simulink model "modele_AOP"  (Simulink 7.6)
settings: Solver=ode45  StartTime=0.0  StopTime=10.0  RelTol=1e-3
InitFcn:
  | Ad=10^5;
  | Vsat=15;
libraries: fl_lib x18

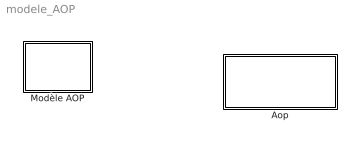
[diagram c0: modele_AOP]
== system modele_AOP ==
  Aop : Subsystem
  Modèle AOP : Subsystem

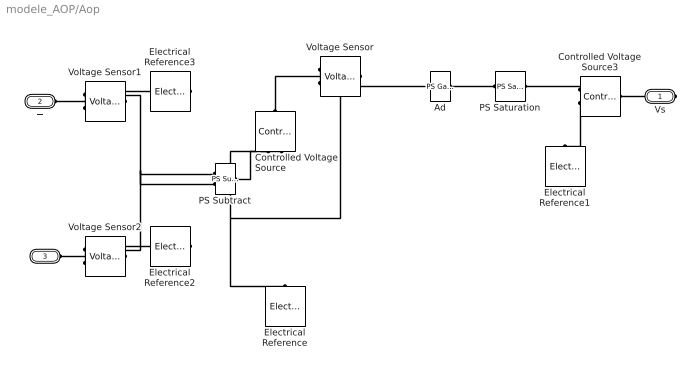
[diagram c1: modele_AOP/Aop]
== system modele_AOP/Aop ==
  Ad : fl_lib/Physical Signals/Functions/PS Gain  DialogController=NetworkEngine.DynNeDlgSource  SystemSampleTime=-1  gain=Ad  LocalVarLogging=[]
  Controlled Voltage Source : fl_lib/Electrical/Electrical Sources/Controlled Voltage Source  DialogController=NetworkEngine.DynNeDlgSource  SystemSampleTime=-1  i_Log=off  v_Log=off  LocalVarNames=|i|v  LocalVarDescs=|i|v  LocalVarLogging=[0 0]
  Controlled Voltage Source3 : fl_lib/Electrical/Electrical Sources/Controlled Voltage Source  DialogController=NetworkEngine.DynNeDlgSource  SystemSampleTime=-1  i_Log=off  v_Log=off  LocalVarNames=|i|v  LocalVarDescs=|i|v  LocalVarLogging=[0 0]
  Electrical Reference{,1..3} (4 alike) : fl_lib/Electrical/Electrical Elements/Electrical Reference  DialogController=NetworkEngine.DynNeDlgSource  SystemSampleTime=-1  i_Log=off  LocalVarNames=|i  LocalVarDescs=|i  LocalVarLogging=0
  PS Saturation : fl_lib/Physical Signals/Nonlinear Operators/PS Saturation  DialogController=NetworkEngine.DynNeDlgSource  SystemSampleTime=-1  upper_limit=Vsat  lower_limit=-Vsat  LocalVarLogging=[]
  PS Subtract : fl_lib/Physical Signals/Functions/PS Subtract  DialogController=NetworkEngine.DynNeDlgSource  SystemSampleTime=-1  LocalVarLogging=[]
  Voltage Sensor : fl_lib/Electrical/Electrical Sensors/Voltage Sensor  DialogController=NetworkEngine.DynNeDlgSource  SystemSampleTime=-1  i1_Log=off  v1_Log=off  LocalVarNames=|i1|v1  LocalVarDescs=|i1|v1  LocalVarLogging=[0 0]
  Voltage Sensor1 : fl_lib/Electrical/Electrical Sensors/Voltage Sensor  DialogController=NetworkEngine.DynNeDlgSource  SystemSampleTime=-1  i1_Log=off  v1_Log=off  LocalVarNames=|i1|v1  LocalVarDescs=|i1|v1  LocalVarLogging=[0 0]
  Voltage Sensor2 : fl_lib/Electrical/Electrical Sensors/Voltage Sensor  DialogController=NetworkEngine.DynNeDlgSource  SystemSampleTime=-1  i1_Log=off  v1_Log=off  LocalVarNames=|i1|v1  LocalVarDescs=|i1|v1  LocalVarLogging=[0 0]
  Vs : PMIOPort  Port=1  Side=Right
  + : PMIOPort  Port=2  Side=Left
  - : PMIOPort  Port=3  Side=Left
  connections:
  Voltage Sensor/RConn1 -- Ad/LConn1
  PS Saturation/LConn1 -- Ad/RConn1
  Controlled Voltage Source/LConn1 -- Voltage Sensor/LConn1
  PS Subtract/RConn1 -- Controlled Voltage Source/RConn1
  Voltage Sensor/RConn2 -- Electrical Reference/LConn1 -- Controlled Voltage Source/RConn2
  Controlled Voltage Source3/RConn1 -- PS Saturation/RConn1
  Controlled Voltage Source3/RConn2 -- Electrical Reference1/LConn1
  Vs/RConn1 -- Controlled Voltage Source3/LConn1
  +/RConn1 -- Voltage Sensor1/LConn1
  -/RConn1 -- Voltage Sensor2/LConn1
  Voltage Sensor2/RConn1 -- PS Subtract/LConn2
  Voltage Sensor1/RConn1 -- PS Subtract/LConn1
  Voltage Sensor1/RConn2 -- Electrical Reference3/LConn1
  Voltage Sensor2/RConn2 -- Electrical Reference2/LConn1

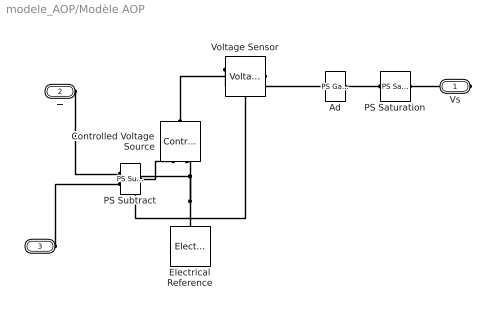
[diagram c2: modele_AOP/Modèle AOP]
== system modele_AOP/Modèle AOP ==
  Ad : fl_lib/Physical Signals/Functions/PS Gain  DialogController=NetworkEngine.DynNeDlgSource  SystemSampleTime=-1  gain=Ad  LocalVarLogging=[]
  Controlled Voltage Source : fl_lib/Electrical/Electrical Sources/Controlled Voltage Source  DialogController=NetworkEngine.DynNeDlgSource  SystemSampleTime=-1  i_Log=off  v_Log=off  LocalVarNames=|i|v  LocalVarDescs=|i|v  LocalVarLogging=[0 0]
  Electrical Reference : fl_lib/Electrical/Electrical Elements/Electrical Reference  DialogController=NetworkEngine.DynNeDlgSource  SystemSampleTime=-1  i_Log=off  LocalVarNames=|i  LocalVarDescs=|i  LocalVarLogging=0
  PS Saturation : fl_lib/Physical Signals/Nonlinear Operators/PS Saturation  DialogController=NetworkEngine.DynNeDlgSource  SystemSampleTime=-1  upper_limit=Vsat  lower_limit=-Vsat  LocalVarLogging=[]
  PS Subtract : fl_lib/Physical Signals/Functions/PS Subtract  DialogController=NetworkEngine.DynNeDlgSource  SystemSampleTime=-1  LocalVarLogging=[]
  Voltage Sensor : fl_lib/Electrical/Electrical Sensors/Voltage Sensor  DialogController=NetworkEngine.DynNeDlgSource  SystemSampleTime=-1  i1_Log=off  v1_Log=off  LocalVarNames=|i1|v1  LocalVarDescs=|i1|v1  LocalVarLogging=[0 0]
  Vs : PMIOPort  Port=1  Side=Right
  + : PMIOPort  Port=2  Side=Left
  - : PMIOPort  Port=3  Side=Left
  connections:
  Voltage Sensor/RConn1 -- Ad/LConn1
  PS Saturation/LConn1 -- Ad/RConn1
  Controlled Voltage Source/LConn1 -- Voltage Sensor/LConn1
  PS Subtract/RConn1 -- Controlled Voltage Source/RConn1
  Controlled Voltage Source/RConn2 -- Electrical Reference/LConn1 -- Voltage Sensor/RConn2
  Vs/RConn1 -- PS Saturation/RConn1
  +/RConn1 -- PS Subtract/LConn1
  -/RConn1 -- PS Subtract/LConn2
